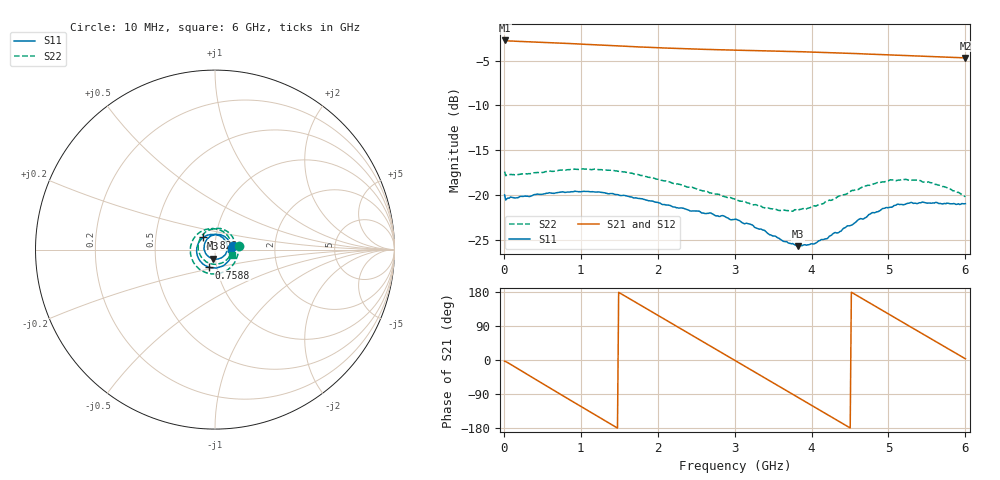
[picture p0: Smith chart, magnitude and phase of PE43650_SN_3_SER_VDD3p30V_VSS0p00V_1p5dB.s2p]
!Keysight Technologies,N5245B,MY57181451,A.13.50.07
!Date: Tuesday, May 07, 2019 07:59:47
!Correction: S11(Full 2 Port(1,2))
!S21(Full 2 Port(1,2))
!S12(Full 2 Port(1,2))
!S22(Full 2 Port(1,2))
!S2P File: Measurements: S11, S21, S12, S22:
# Hz S  dB  R 50
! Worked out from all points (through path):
!   401 points, 10 MHz to 6 GHz, reference 50 ohm
!   highest |S21| = -2.73 dB at 10 MHz (marker M1); lowest = -4.7 dB at 6 GHz (marker M2)
!   group delay of S21, straight-line fit = 331 ps
!   lowest |S11| = -25.7 dB at 3.829 GHz (marker M3), VSWR 1.11, Z = 48.8 - j4.98 ohm
!   |S11| at or under -10 dB: start of sweep to end of sweep
!   |S22| runs from -21.8 to -17.1 dB; largest |S21 - S12| = 0.0052
!   S11 on the Smith chart (normalised r, x): 10 MHz: 1.22, +0.05; 758.8 MHz: 0.92, -0.18; 1.822 GHz: 0.87, +0.12; 6 GHz: 1.20, +0.01
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1e7  -19.99 12.6  -2.73 -3.3  -2.79 -3.2  -17.39 9.1
2.04675e8  -20.19 -30.5  -2.84 -25.8  -2.89 -25.8  -17.69 -30.2
4.293e8  -19.91 -63.3  -2.92 -53.2  -2.97 -53.2  -17.49 -62.4
7.5875e8  -19.65 -107.7  -3.04 -93.2  -3.09 -93.2  -17.20 -107.4
1.013325e9  -19.62 -140.2  -3.15 -124.0  -3.20 -124.0  -17.10 -140.0
1.41765e9  -19.85 174.2  -3.31 -172.5  -3.37 -172.5  -17.25 173.0
1.821975e9  -20.50 134.2  -3.48 139.3  -3.54 139.3  -17.86 129.6
2.01665e9  -20.88 116.6  -3.55 116.2  -3.60 116.2  -18.26 110.0
2.241275e9  -21.42 96.7  -3.63 89.5  -3.68 89.5  -18.78 87.4
2.4659e9  -21.78 75.9  -3.69 62.9  -3.75 62.9  -19.20 64.5
2.750425e9  -22.32 49.6  -3.76 29.2  -3.82 29.3  -19.90 34.1
3.005e9  -22.71 20.8  -3.81 -1.0  -3.87 -0.9  -20.47 4.6
3.45425e9  -24.44 -37.8  -3.91 -54.4  -3.95 -54.3  -21.50 -57.9
3.828625e9  -25.72 -100.5  -3.99 -99.0  -4.03 -98.9  -21.69 -116.6
4.008325e9  -25.46 -134.0  -4.02 -120.4  -4.07 -120.4  -21.31 -146.0
4.2629e9  -24.46 -178.7  -4.10 -150.8  -4.15 -150.7  -20.58 174.8
4.5025e9  -23.42 144.8  -4.17 -179.4  -4.23 -179.2  -19.63 140.4
4.7421e9  -22.20 112.2  -4.26 152.1  -4.31 152.2  -18.91 109.7
5.01165e9  -21.39 81.7  -4.35 120.1  -4.40 120.3  -18.35 77.2
5.445925e9  -20.78 40.1  -4.50 68.7  -4.55 68.8  -18.56 30.8
5.745425e9  -20.98 18.5  -4.60 33.3  -4.65 33.4  -19.14 2.6
6e9  -20.97 3.1  -4.68 3.2  -4.73 3.3  -20.20 -18.5
